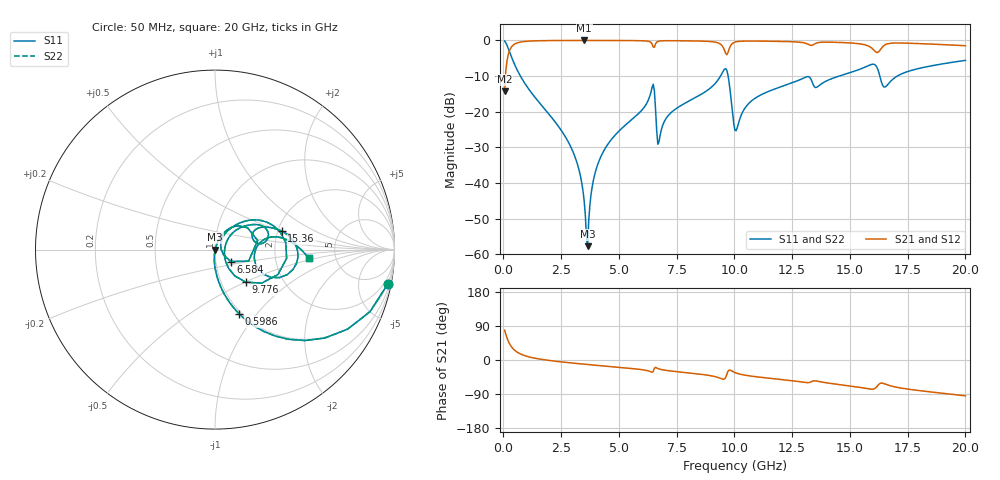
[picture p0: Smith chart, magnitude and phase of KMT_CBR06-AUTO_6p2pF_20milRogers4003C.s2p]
! Data measured by Modelithics Inc. support@modelithics.com 813-866-6335
! KEMET CBR06-AUTO 6.2pF, Pad Width= 0.851mm, Pad Length= 0.64mm, Pad Gap= 0.62mm, 20mil Rogers 4003C substrate Data, January 2022
# hz S ma R 50
! 2 Port Network Data from SP1.SP block
! freq  magS11  angS11  magS21  angS21  magS12  angS12  magS22  angS22
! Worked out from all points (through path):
!   401 points, 50 MHz to 20 GHz, reference 50 ohm
!   highest |S21| = -0.01 dB at 3.491 GHz (marker M1); lowest = -14.3 dB at 50 MHz (marker M2)
!   group delay of S21, straight-line fit = 14.6 ps
!   lowest |S11| = -57.7 dB at 3.641 GHz (marker M3), VSWR 1.00, Z = 50.1 + j0.0384 ohm
!   |S11| at or under -10 dB: 733.6 MHz to 9.398 GHz (8.664 GHz wide, 171 % of centre); 9.728 GHz to 14.54 GHz (4.811 GHz wide, 39.7 % of centre); 16.3 GHz to 17.05 GHz (755.9 MHz wide, 4.53 % of centre)
!   |S22| runs from -57.7 to -0.2 dB; largest |S21 - S12| = 0
!   S11 on the Smith chart (normalised r, x): 50 MHz: 1, -10; 598.6 MHz: 0.97, -0.82; 6.584 GHz: 1.18, -0.16; 9.776 GHz: 1.30, -0.50; 15.36 GHz: 2.11, +0.51; 20 GHz: 3.15, -0.42
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5e7  0.9812 -11.3  0.1929 78.7  0.1929 78.7  0.9812 -11.3
2.495e8  0.7121 -45.4  0.7015 44.6  0.7015 44.6  0.7121 -45.4
5.98625e8  0.3824 -69.4  0.9234 20.5  0.9234 20.5  0.3824 -69.4
2.74325e9  0.04103 -95.2  0.9981 -6.6  0.9981 -6.6  0.04103 -95.2
3.391625e9  0.009971 -94.2  0.9987 -10.5  0.9987 -10.5  0.009971 -94.2
3.491375e9  0.005733 -89.9  0.9988 -11.0  0.9988 -11.0  0.005733 -89.9
3.641e9  0.001298 17.2  0.9987 -11.9  0.9987 -11.9  0.001298 17.2
3.94025e9  0.01271 71.1  0.9986 -13.5  0.9986 -13.5  0.01271 71.1
4.389125e9  0.02997 71.5  0.9981 -16.0  0.9981 -16.0  0.02997 71.5
6.434e9  0.2183 33.8  0.8916 -32.4  0.8916 -32.4  0.2183 33.8
6.583625e9  0.1101 -37.1  0.8943 -19.4  0.8943 -19.4  0.1101 -37.1
6.73325e9  0.03775 31.9  0.9779 -23.6  0.9779 -23.6  0.03775 31.9
9.32675e9  0.2901 34.6  0.914 -46.7  0.914 -46.7  0.2901 34.6
9.626e9  0.4019 -7.0  0.6533 -45.5  0.6533 -45.5  0.4019 -7.0
9.775625e9  0.2487 -46.8  0.7626 -26.5  0.7626 -26.5  0.2487 -46.8
1.0025e10  0.05471 -16.2  0.9472 -33.2  0.9472 -33.2  0.05471 -16.2
1.107238e10  0.1672 42.3  0.9781 -45.2  0.9781 -45.2  0.1672 42.3
1.336662e10  0.2608 7.2  0.855 -56.2  0.855 -56.2  0.2608 7.2
1.536162e10  0.3865 15.4  0.9008 -71.5  0.9008 -71.5  0.3865 15.4
1.62095e10  0.3923 -23.4  0.6784 -67.1  0.6784 -67.1  0.3923 -23.4
1.670825e10  0.2554 9.0  0.9076 -67.3  0.9076 -67.3  0.2554 9.0
2e10  0.5249 -5.3  0.8425 -94.5  0.8425 -94.5  0.5249 -5.3
